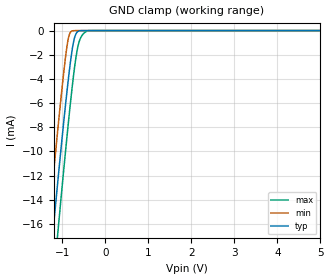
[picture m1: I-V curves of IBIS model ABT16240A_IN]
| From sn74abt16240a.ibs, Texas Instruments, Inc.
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[Model]   ABT16240A_IN
Model_type  Input
Vinl = 0.8
Vinh = 2.0
| variable   typ   min   max
C_comp   2.07pF   1.64pF   3.12pF
[Temperature Range]   40   -40   100
| Ambient temperature   25   -40   85
[Voltage range]   5   4.5   5.5
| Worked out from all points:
|   GND clamp passes 1 mA (typ) near -0.74 V on its own axis
[GND Clamp]
| ABT16240A_IN
|   Voltage   I(typ)   I(min)   I(max)
-5V       -198.1mA   -179.5mA   -207.8mA
-1.375V   -23.32mA   -18.47mA   -28.66mA
-1.315V   -20.66mA   -16.16mA   -25.81mA
-1.215V   -16.78mA   -12.39mA   -21.26mA
-1.095V   -12.29mA   -7.993mA   -16.55mA
-895mV    -5.273mA   -1.497mA   -9.049mA
-840mV    -3.546mA   -422.7uA   -7.11mA
-775mV    -1.773mA   -45.42uA   -4.946mA
-705mV    -511.6uA   -2.645uA   -2.881mA
-615mV    -36.14uA   -37.52nA   -1.049mA
-410mV    -25.44nA   -45.74pA   -21.15uA
5V        88.45pA    93.15pA    937.5pA
